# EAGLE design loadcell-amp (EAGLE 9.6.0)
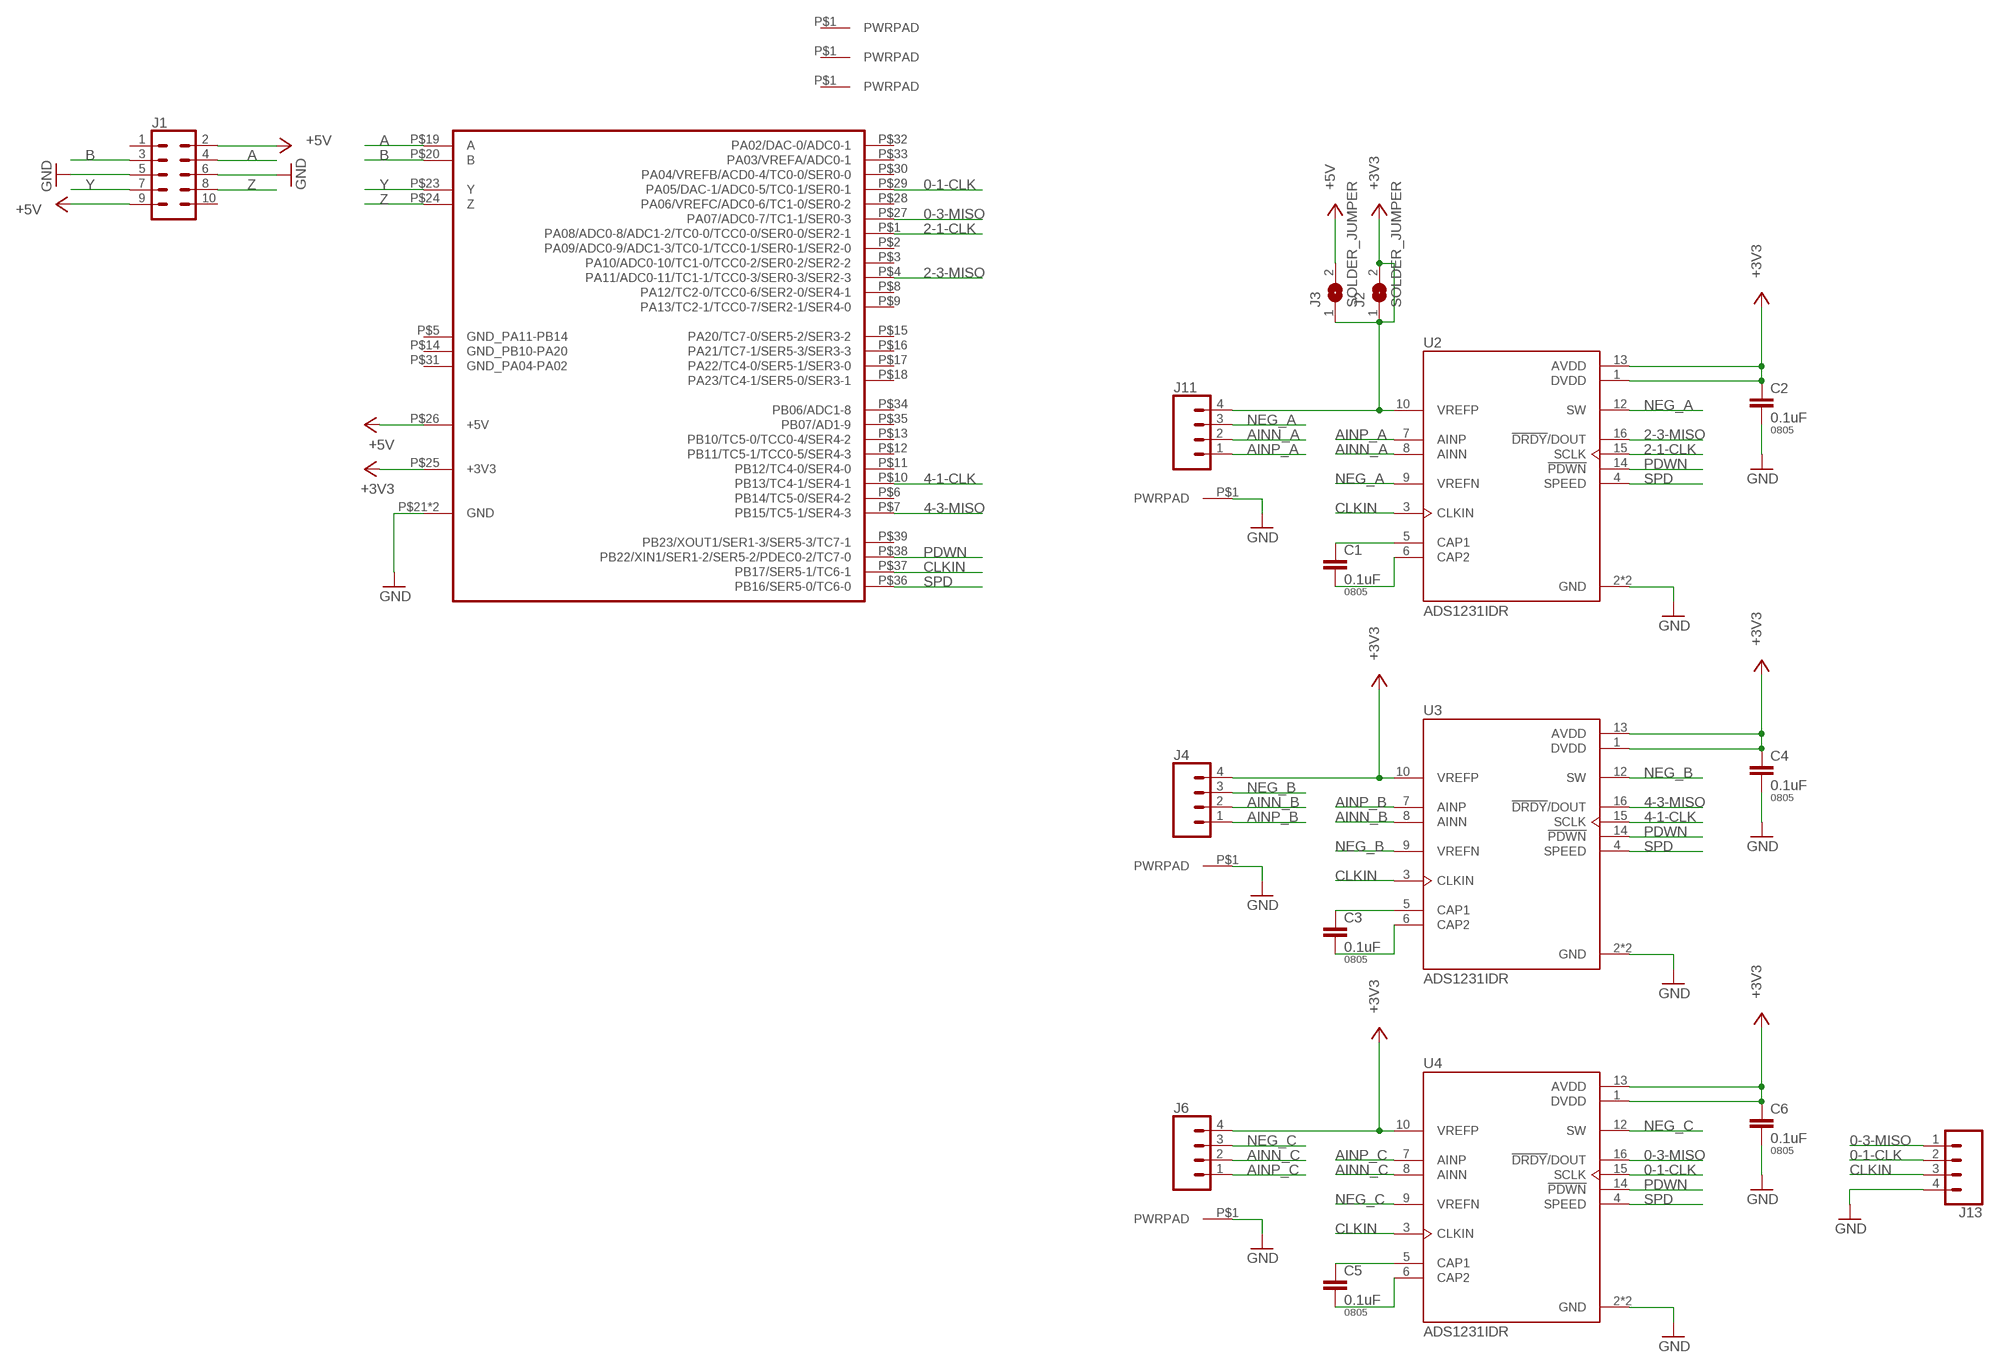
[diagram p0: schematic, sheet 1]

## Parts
C1  0.1uF  CAP0805  [0805]
C2  0.1uF  CAP0805  [0805]
C3  0.1uF  CAP0805  [0805]
C4  0.1uF  CAP0805  [0805]
C5  0.1uF  CAP0805  [0805]
C6  0.1uF  CAP0805  [0805]
J1  CONN_05X2SHD_LOCK_LATCH  [2X5-SHROUDED_LOCK_LATCH]
J2  SOLDER_JUMPER  [SOLDER_JUMPER]
J3  SOLDER_JUMPER  [SOLDER_JUMPER]
J4  CONN_04LOCK_LONGPADS  [1X04_LOCK_LONGPADS]
J5  PWRPADSOLDER_SMALL  [SOLDER_ON_SMALL]
J6  CONN_04LOCK_LONGPADS  [1X04_LOCK_LONGPADS]
J7  PWRPADSOLDER_SMALL  [SOLDER_ON_SMALL]
J8  PWRPADM3  [PWRPAD_3-25MM]
J9  PWRPADM3  [PWRPAD_3-25MM]
J10  PWRPADM3  [PWRPAD_3-25MM]
J11  CONN_04LOCK_LONGPADS  [1X04_LOCK_LONGPADS]
J12  PWRPADSOLDER_SMALL  [SOLDER_ON_SMALL]
J13  CONN_04LOCK  [1X04_LOCK]
U1  UCBUS_MODULE_EXT  [UCBUS_MODULE_EXT]
U2  ADS1231IDR  [SOIC127P600X175-16N]
U3  ADS1231IDR  [SOIC127P600X175-16N]
U4  ADS1231IDR  [SOIC127P600X175-16N]

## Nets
0-1-CLK: J13.2 U1.P$29(PA05/DAC-1/ADC0-5/TC0-1/SER0-1) U4.15(SCLK)
0-3-MISO: J13.1 U1.P$27(PA07/ADC0-7/TC1-1/SER0-3) U4.16(!DRDY!/DOUT)
2-1-CLK: U1.P$1(PA08/ADC0-8/ADC1-2/TC0-0/TCC0-0/SER0-0/SER2-1) U2.15(SCLK)
2-3-MISO: U1.P$4(PA11/ADC0-11/TC1-1/TCC0-3/SER0-3/SER2-3) U2.16(!DRDY!/DOUT)
4-1-CLK: U1.P$10(PB13/TC4-1/SER4-1) U3.15(SCLK)
4-3-MISO: U1.P$7(PB15/TC5-1/SER4-3) U3.16(!DRDY!/DOUT)
+3V3: C2.1 C4.1 C6.1 J2.1 J2.2 J3.1 J4.4 J6.4 J11.4 U1.P$25(+3V3) U2.1(DVDD) U2.10(VREFP) U2.13(AVDD) U3.1(DVDD) U3.10(VREFP) U3.13(AVDD) U4.1(DVDD) U4.10(VREFP) U4.13(AVDD)
+5V: J1.2 J1.9 J3.2 U1.P$26(+5V)
A: J1.4 U1.P$19(A)
AINN_A: J11.2 U2.8(AINN)
AINN_B: J4.2 U3.8(AINN)
AINN_C: J6.2 U4.8(AINN)
AINP_A: J11.1 U2.7(AINP)
AINP_B: J4.1 U3.7(AINP)
AINP_C: J6.1 U4.7(AINP)
B: J1.3 U1.P$20(B)
CLKIN: J13.3 U1.P$37(PB17/SER5-1/TC6-1) U2.3(CLKIN) U3.3(CLKIN) U4.3(CLKIN)
GND: C2.2 C4.2 C6.2 J1.5 J1.6 J5.P$1(PWRPAD) J7.P$1(PWRPAD) J12.P$1(PWRPAD) J13.4 U1.P$21(GND) U1.P$22(GND) U2.2(GND) U2.11(GND) U3.2(GND) U3.11(GND) U4.2(GND) U4.11(GND)
N$1: C1.1 U2.5(CAP1)
N$2: C3.1 U3.5(CAP1)
N$3: C3.2 U3.6(CAP2)
N$4: C1.2 U2.6(CAP2)
N$5: C5.1 U4.5(CAP1)
N$6: C5.2 U4.6(CAP2)
NEG_A: J11.3 U2.9(VREFN) U2.12(SW)
NEG_B: J4.3 U3.9(VREFN) U3.12(SW)
NEG_C: J6.3 U4.9(VREFN) U4.12(SW)
PDWN: U1.P$38(PB22/XIN1/SER1-2/SER5-2/PDEC0-2/TC7-0) U2.14(!PDWN) U3.14(!PDWN) U4.14(!PDWN)
SPD: U1.P$36(PB16/SER5-0/TC6-0) U2.4(SPEED) U3.4(SPEED) U4.4(SPEED)
Y: J1.7 U1.P$23(Y)
Z: J1.8 U1.P$24(Z)
Unconnected: J1.1 J1.10 J8.P$1(PWRPAD) J9.P$1(PWRPAD) J10.P$1(PWRPAD) U1.P$2(PA09/ADC0-9/ADC1-3/TC0-1/TCC0-1/SER0-1/SER2-0) U1.P$3(PA10/ADC0-10/TC1-0/TCC0-2/SER0-2/SER2-2) U1.P$5(GND_PA11-PB14) U1.P$6(PB14/TC5-0/SER4-2) U1.P$8(PA12/TC2-0/TCC0-6/SER2-0/SER4-1) U1.P$9(PA13/TC2-1/TCC0-7/SER2-1/SER4-0) U1.P$11(PB12/TC4-0/SER4-0) U1.P$12(PB11/TC5-1/TCC0-5/SER4-3) U1.P$13(PB10/TC5-0/TCC0-4/SER4-2) U1.P$14(GND_PB10-PA20) U1.P$15(PA20/TC7-0/SER5-2/SER3-2) U1.P$16(PA21/TC7-1/SER5-3/SER3-3) U1.P$17(PA22/TC4-0/SER5-1/SER3-0) U1.P$18(PA23/TC4-1/SER5-0/SER3-1) U1.P$28(PA06/VREFC/ADC0-6/TC1-0/SER0-2) U1.P$30(PA04/VREFB/ACD0-4/TC0-0/SER0-0) U1.P$31(GND_PA04-PA02) U1.P$32(PA02/DAC-0/ADC0-1) U1.P$33(PA03/VREFA/ADC0-1) U1.P$34(PB06/ADC1-8) U1.P$35(PB07/AD1-9) U1.P$39(PB23/XOUT1/SER1-3/SER5-3/TC7-1)

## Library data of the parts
C1-C6 = passives:CAP: Capacitor; PACKAGE: 0805
J1 = SparkFun-Connectors:CONN_05X2: Multi connection point. Often used as Generic Header-pin footprint for 0.1 inch spaced/style header connections For AVR SPI programming port, see special device with nice symbol: "AVR_SPI_PROG_5x2.dev" You can populate with any combo of single row headers, but if you'd like an exact match, check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
J2 J3 = connector:SOLDER_JUMPER
J4 J6 J11 J13 = SparkFun-Connectors:CONN_04: Multi connection point. Often used as Generic Header-pin footprint for 0.1 inch spaced/style header connections On any of the 0.1 inch spaced packages, you can populate with these: Break Away Headers - Straight (PRT-00116) Break Away Male Headers - Right Angle (PRT-00553) Female Headers (PRT-00115)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; PROD_ID: CONN-09696
J5 J7-J10 J12 = connector:PWRPAD
U1 = connector:UCBUS_MODULE_EXT
U2-U4 = sensor:ADS1231IDR: 24-Bit, 80SPS, 1-Ch Delta-Sigma ADC for Resistive Bridge Sensors & Weigh Scales 16-SOIC -40 to 85 Check prices; AVAILABILITY: Good; DESCRIPTION: 24-Bit, 80SPS, 1-Ch Delta-Sigma ADC for Resistive Bridge Sensors & Weigh Scales 16-SOIC -40 to 85; MF: Texas Instruments; MP: ADS1231IDR; PACKAGE: SOIC-16 Texas Instruments; PRICE: None; PURCHASE-URL: https://pricing.snapeda.com/search/part/ADS1231IDR/?ref=eda

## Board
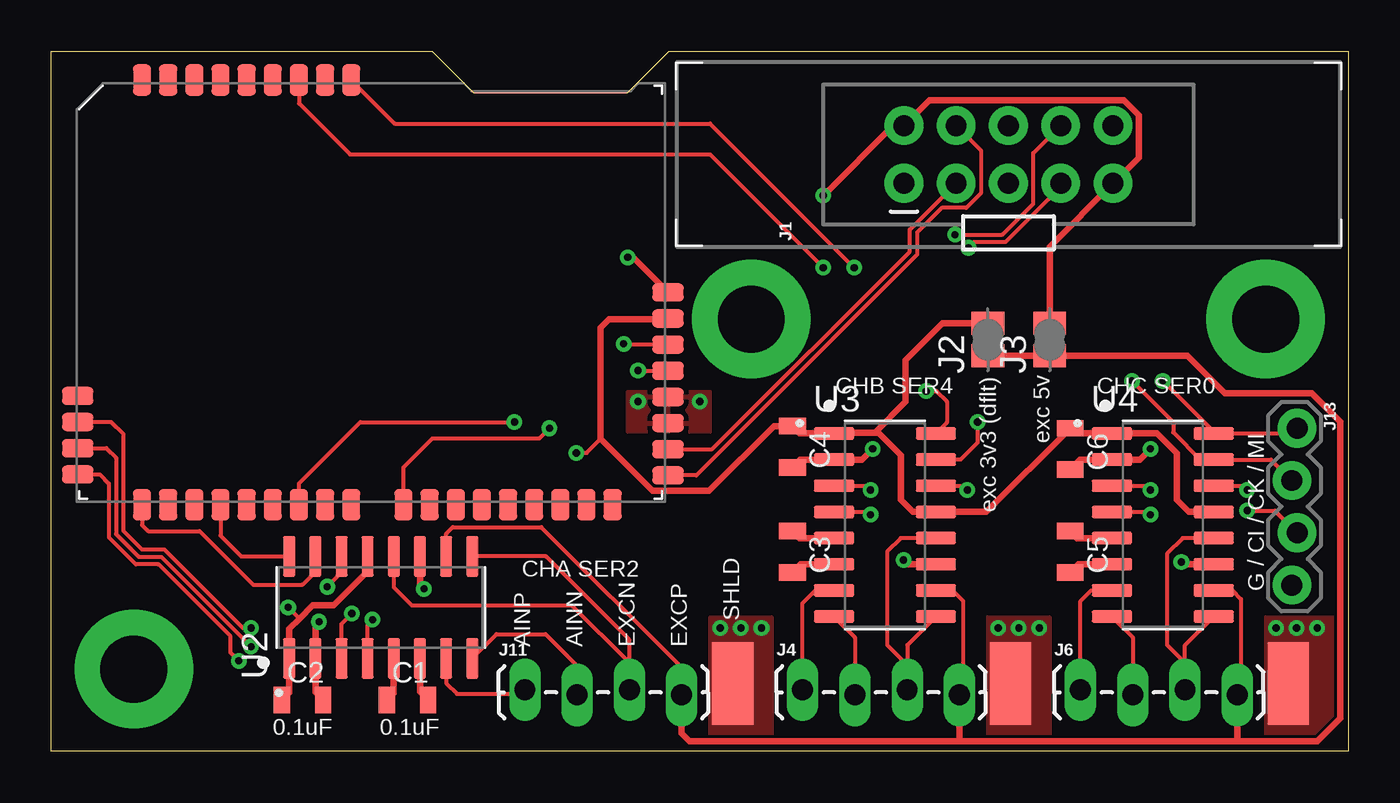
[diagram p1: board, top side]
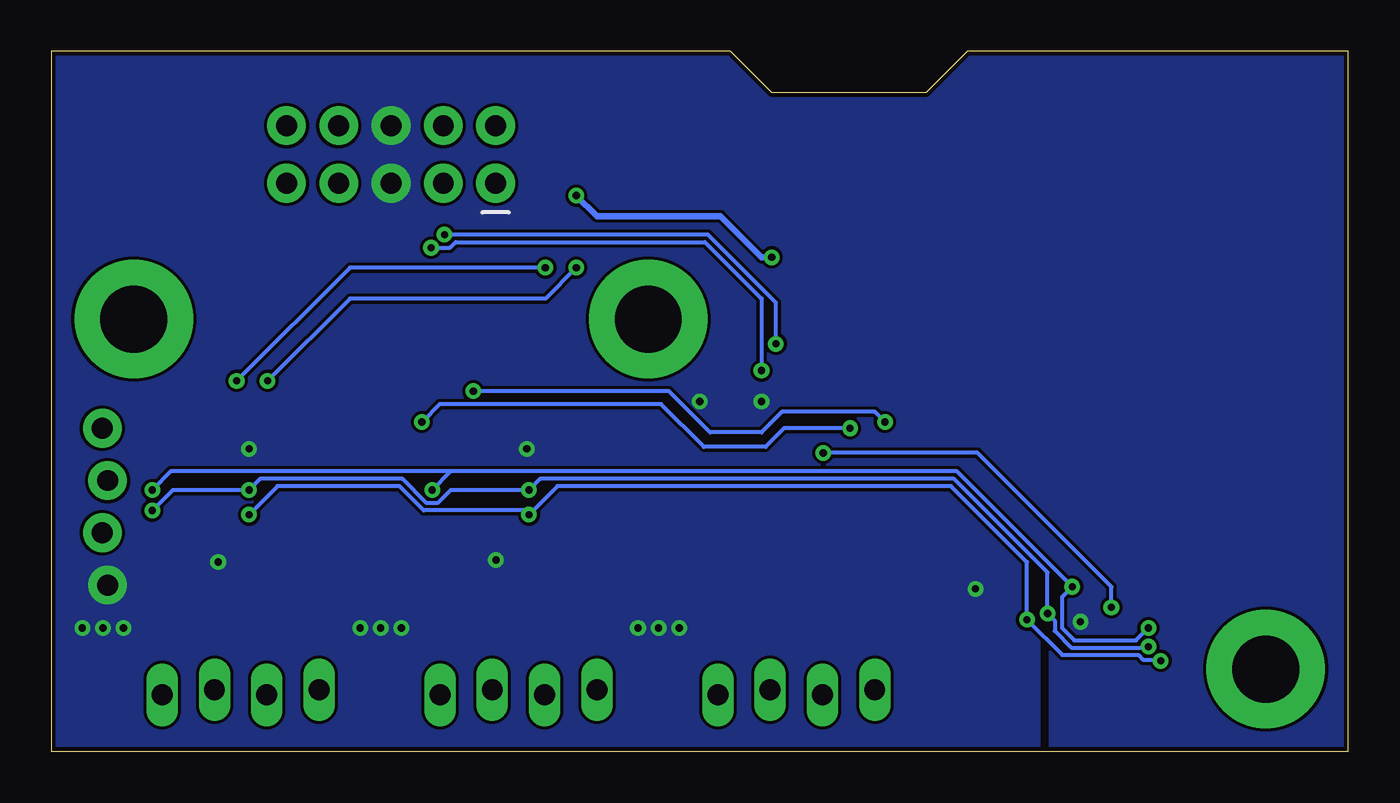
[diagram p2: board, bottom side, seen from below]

Size 63 x 34 mm. Coordinates in mm from the lower left corner, seen from the top.
Outline: 0,0 0,34 18.5,34 20.5,32 28,32 30,34 63,34 63,0 0,0
Copper layers (1*16): Top 0.035mm / dielectric 1.5mm / Bottom 0.035mm
Design rules "default *": minimum track width 6mil, minimum drill 0.35mm, track to track 6mil, track to pad 6mil, pad to pad 6mil, via to via 6mil, smd to smd 6mil, copper to edge 8mil, drill to drill 6mil, minimum pad ring 10mil, minimum via ring 8mil, stop-mask expansion 4mil, vias tented up to drill 35mil, thermal gap 10mil

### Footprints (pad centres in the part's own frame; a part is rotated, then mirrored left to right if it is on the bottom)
0805 = smd 0.8 x 1.3: 1 -1,0; 2 1,0
2X5-SHROUDED_LOCK_LATCH = drill 1.016 pad 1.88: 1 -1.397,5.08; 2 1.397,5.08; 3 -1.397,2.54; 4 1.397,2.54; 5 -1.397,0; 6 1.397,0; 7 -1.397,-2.54; 8 1.397,-2.54; 9 -1.397,-5.08; 10 1.397,-5.08
SOLDER_JUMPER = smd 1.118 x 1.6: 1 -0.787,0; 2 0.787,0
1X04_LOCK_LONGPADS = drill 1.016 long: 1 0,0; 2 2.54,-0.254; 3 5.08,0; 4 7.62,-0.254
SOLDER_ON_SMALL = smd 2 x 4: P$1 0,0
PWRPAD_3-25MM = drill 3.25 pad 5.75: P$1 0,0
1X04_LOCK = drill 1.016 pad 1.88: 1 0,0.127; 2 2.54,-0.127; 3 5.08,0.127; 4 7.62,-0.127
UCBUS_MODULE_EXT = smd 0.889 x 1.524: P$1 3.175,-0.152; P$2 4.445,-0.152; P$3 5.715,-0.152; P$4 6.985,-0.152; P$5 8.255,-0.152; P$6 9.525,-0.152; P$7 10.795,-0.152; P$8 12.065,-0.152; P$9 13.335,-0.152; P$10 15.875,-0.152; P$11 17.145,-0.152; P$12 18.415,-0.152; P$13 19.685,-0.152; P$14 20.955,-0.152; P$15 22.225,-0.152; P$16 23.495,-0.152; P$17 24.765,-0.152; P$18 26.035,-0.152; P$27 13.335,20.472; P$28 12.065,20.472; P$29 10.795,20.472; P$30 9.525,20.472; P$31 8.255,20.472; P$32 6.985,20.472; P$33 5.715,20.472; P$34 4.445,20.472; P$35 3.175,20.472 | smd 1.524 x 0.889: P$19 28.727,1.27; P$20 28.727,2.54; P$21 28.727,3.81; P$22 28.727,5.08; P$23 28.727,6.35; P$24 28.727,7.62; P$25 28.727,8.89; P$26 28.727,10.16; P$36 0.05,1.32; P$37 0.05,2.59; P$38 0.05,3.86; P$39 0.05,5.13
SOIC127P600X175-16N = smd 1.97 x 0.6: 1 -2.475,4.445; 2 -2.475,3.175; 3 -2.475,1.905; 4 -2.475,0.635; 5 -2.475,-0.635; 6 -2.475,-1.905; 7 -2.475,-3.175; 8 -2.475,-4.445; 9 2.475,-4.445; 10 2.475,-3.175; 11 2.475,-1.905; 12 2.475,-0.635; 13 2.475,0.635; 14 2.475,1.905; 15 2.475,3.175; 16 2.475,4.445

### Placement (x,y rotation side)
C1  17.3,2.5 0 top
C2  12.2,2.5 0 top
C3  36,9.7 270 top
C4  36,14.8 270 top
C5  49.5,9.7 270 top
C6  49.5,14.7 270 top
J1  46.5,29 90 top
J2  45.5,20 90 top
J3  48.5,20 90 top
J4  36.5,3 0 top
J5  46.6,3.3 0 top
J6  50,3 0 top
J7  60.1,3.3 0 top
J8  4,4 0 top
J9  59,21 0 top
J10  34,21 0 top
J11  23,3 0 top
J12  33.1,3.3 0 top
J13  60.4,15.7 270 top
U1  1.23,12.14 0 top
U2  16,7 90 top
U3  40.5,11 0 top
U4  54,11 0 top

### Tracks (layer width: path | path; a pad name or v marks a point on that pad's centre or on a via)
0-1-CLK  (via drill 0.35)
  Top 0.203: U1.P$29 12.03,31.48 14.5,29 32,29 v37.5,23.5 | v52.5,18 54.5,16 54.5,15.5 55.83,14.18 U4.15 59.26,14.18 J13.2
  Bottom 0.203: v37.5,23.5 39,22 48.5,22 v52.5,18
0-3-MISO  (via drill 0.35)
  Top 0.203: U1.P$27 16.68,30.5 32,30.5 v39,23.5 | v54,18 56.48,15.53 U4.16 60.27,15.45 J13.1
  Bottom 0.203: v39,23.5 48.5,23.5 v54,18
2-1-CLK
  Top 0.203: U1.P$1 4.41,10.99 4.7,10.7 7.2,10.7 9.8,8.1 12.2,8.1 12.82,8.72 U2.15
2-3-MISO
  Top 0.203: U1.P$4 8.21,10.48 9.22,9.47 U2.16
4-1-CLK  (via drill 0.35)
  Top 0.203: U1.P$10 17.11,13.8 18.5,15.2 23.7,15.2 v24.2,15.7 | v45,16 45,15 44.17,14.18 U3.15
  Bottom 0.203: v24.2,15.7 27.4,15.7 28.3,14.8 31.3,14.8 33.37,16.87 42.23,16.87 42.24,16.87 44.13,16.87 v45,16
4-3-MISO  (via drill 0.35)
  Top 0.203: U1.P$7 12.03,13.03 15,16 v22.5,16 | v42.5,17.5 43,17.5 43.5,17 43.5,15.97 U3.16
  Bottom 0.203: v22.5,16 23,16.5 27.5,16.5 28.5,15.5 31,15.5 33,17.5 v42.5,17.5
+3V3  (via drill 0.35)
  Top 0.203: J11.4 30.62,4.08 23.8,10.9 19.5,10.9 19.18,10.57 U2.10 | U3.10 43.77,7.83 44.3,7.3 44.3,4 44.12,3.82 J4.4 | U4.10 57.38,7.83 57.8,7.4 57.8,2.93 J6.4 | J2.1 J2.2 | 12.05,6.45 v11.5,7 | v25.5,14.5 26,14.5 26.68,15.18
  Top 0.305: U2.13 15.37,8.77 13.7,7.1 12.7,7.1 12.05,6.45 11.55,5.96 U2.1 11.55,2.85 C2.1 | 40,15.48 38.06,15.48 U3.1 36.35,15.45 C4.1 35.1,15.8 31.96,12.66 29.2,12.66 26.68,15.18 26.68,20.58 27.1,21 29.93,21 U1.P$25 | 40,15.48 40.19,15.48 41.28,14.38 41.28,12.22 41.87,11.63 U3.13 45.44,11.63 C6.1 49.76,15.45 U4.1 53.72,15.45 54.68,14.48 54.68,12.22 55.27,11.63 U4.13 | J2.1 J3.1 55.19,19.21 57,17.4 61.24,17.4 62.62,16.02 62.62,1.62 61.5,0.5 57.5,0.5 | 57.5,0.5 44,0.5 | 44,0.5 31,0.5 30.62,0.88 J11.4 | J4.4 44.12,0.62 44,0.5 | J6.4 57.62,0.62 57.5,0.5 | 40,15.48 41.5,16.98 41.5,19 43.29,20.79 J2.2
  Bottom 0.203: v11.5,7 11.5,8 18,14.5 v25.5,14.5
+5V  (via drill 0.35)
  Top 0.305: v37.5,27 40.9,30.4 J1.2 42.66,31.64 52.1,31.64 52.83,30.91 52.83,28.85 J1.9 48.5,24.52 J3.2 | v28,24 28.26,24 U1.P$26
  Bottom 0.305: v37.5,27 36.5,26 30.5,26 28.5,24 v28,24
A
  Top 0.203: J1.4 45.15,29.2 45.15,27.11 44.45,26.4 43.26,26.4 42.06,25.2 42.06,24.13 31.34,13.41 U1.P$19
AINN_A
  Top 0.203: U2.8 21.62,5.7 24,5.7 25.54,4.16 J11.2
AINN_B
  Top 0.203: U3.8 39.04,5.54 J4.2
AINN_C
  Top 0.203: U4.8 52.54,5.54 J6.2
AINP_A
  Top 0.203: U2.7 19.18,3.33 19.7,2.8 22.8,2.8 J11.1
AINP_B
  Top 0.203: J4.1 36.5,7.2 37.12,7.83 U3.7
AINP_C
  Top 0.203: J6.1 50,7.3 50.52,7.83 U4.7
B
  Top 0.203: U1.P$20 32.1,14.68 41.7,24.27 41.7,25.34 J1.3
CLKIN  (via drill 0.35)
  Top 0.203: U3.3 39.59,12.9 v39.8,12.7 | U4.3 53.2,12.9 v53.4,12.7 | U2.3 14.1,6.2 v14.6,6.7 | v9.7,5.09 5.35,9.44 4.25,9.44 3.14,10.55 3.14,14.26 2.67,14.73 U1.P$37 | v58.1,11.7 59.45,11.7 J13.3
  Bottom 0.203: v9.7,5.09 9.75,5.04 13.45,5.04 14.26,5.85 14.26,6.36 v14.6,6.7 14.6,8.7 19.15,13.24 39.26,13.24 v39.8,12.7 43.61,12.7 44.24,12.07 44.76,12.07 45.94,13.24 52.86,13.24 v53.4,12.7 57.1,12.7 v58.1,11.7
GND  (via drill 0.35)
  Top 0.305: C2.2 12.82,2.88 U2.2 12.82,6.12 v13,6.3 | C4.2 36.38,14.18 U3.2 39.38,14.18 v39.9,14.7 | C6.2 49.98,14.18 U4.2 52.88,14.18 v53.4,14.7 | U3.11 41.6,9.1 v41.4,9.3 | U4.11 55.01,9.1 v54.9,9.2 | U2.11 17.91,8.1 v18.1,7.9
  other vias: 31.5,17 28.5,17 32.5,6 33.5,6 34.5,6 46,6 47,6 48,6 59.5,6 60.5,6 61.5,6
  pour Bottom (no thermals): -1,36 65,36 65,-1 15,-1 15,7 14.5,7 14.5,-1 -1,-1
  pour Top: 28,17.5 32,17.5 32,15.5 28,15.5
  pour Top (no thermals): 59,6.5 59,-0.5 63.5,-0.5 63.5,6.5
  pour Top (no thermals): 45.5,6.5 45.5,-0.5 48.5,-0.5 48.5,6.5
  pour Top (no thermals): 32,6.5 32,-0.5 35,-0.5 35,6.5
N$1
  Top 0.305: U2.5 16.64,2.83 C1.1
N$2
  Top 0.305: U3.5 36.34,10.37 C3.1
N$3
  Top 0.305: U3.6 36.4,9.1 C3.2
N$4
  Top 0.305: U2.6 17.91,2.9 C1.2
N$5
  Top 0.305: U4.5 49.84,10.37 C5.1
N$6
  Top 0.305: U4.6 49.9,9.1 C5.2
NEG_A
  Top 0.203: U2.12 16.64,7.96 17.5,7.1 25.28,7.1 28.08,4.3 J11.3 28.08,5.42 24.02,9.47 U2.9
NEG_B
  Top 0.203: U3.9 41.58,5.16 41.58,4.2 | 41.58,4.2 J4.3 | U3.12 41.27,10.37 40.6,9.7 40.6,5.18 41.58,4.2
NEG_C
  Top 0.203: J6.3 55.08,4.3 | 55.08,4.3 55.08,5.16 U4.9 | U4.12 54.97,10.37 54.2,9.6 54.2,5.18 55.08,4.3
PDWN  (via drill 0.35)
  Top 0.203: U3.14 44.3,12.9 v44.5,12.7 | U4.14 57.9,12.9 v58.1,12.7 | U2.14 14.1,8.7 v13.4,8 | v9.7,6 9.3,6 5.5,9.8 4.4,9.8 3.5,10.7 3.5,15.4 2.9,16 U1.P$38
  Bottom 0.203: v44.5,12.7 43.6,13.6 | 43.6,13.6 19,13.6 v13.4,8 13.9,7.5 13.9,6 13.3,5.4 10.3,5.4 v9.7,6 | 43.6,13.6 57.2,13.6 v58.1,12.7
SPD  (via drill 0.35)
  Top 0.203: U3.4 39.66,11.63 v39.8,11.5 | U4.4 53.27,11.63 v53.4,11.5 | U2.4 15.37,6.17 v15.6,6.4 | v9.1,4.4 8.7,4.81 8.7,5.59 5.2,9.09 4.11,9.09 2.79,10.4 2.79,13.01 2.34,13.46 U1.P$36
  Bottom 0.203: v53.4,11.5 52.01,12.89 46.09,12.89 44.91,11.71 40.01,11.71 v39.8,11.5 38.41,12.89 19.3,12.89 15.6,9.19 v15.6,6.4 13.89,4.69 10.19,4.69 9.96,4.46 9.16,4.46 v9.1,4.4
Y  (via drill 0.35)
  Top 0.203: J1.7 49.04,27.44 46.35,24.74 44.83,24.74 v44.55,24.47 | v28.5,18.5 29.95,18.5 U1.P$23
  Bottom 0.203: v44.55,24.47 43.64,24.47 43.36,24.74 31.25,24.74 28.5,22 v28.5,18.5
Z  (via drill 0.35)
  Top 0.203: U1.P$24 27.84,19.76 v27.8,19.8 | v43.9,25.1 46.2,25.1 47.7,26.6 47.7,29.06 J1.8
  Bottom 0.203: v27.8,19.8 27.8,21.8 31.1,25.1 v43.9,25.1

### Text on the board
tPlace: CHB SER4 | exc 3v3 (dflt) | exc 5v | CHC SER0 | CHA SER2 | G / CI / CK / MI | SHLD | AINP | AINN | EXCN | EXCP | 0.1uF | 0.1uF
